[IBIS Ver]   2.1
[File Name]   sprm124.ibs
[File Rev]   0.1
[Date]   Sept. 29, 2003
[Source]   IBIS Model Generated from PACED
[Disclaimer]   Please be aware that in the absence of a written agreement
|   Texas Instruments(TI) assumes no liability for:
|   (1) The accuracy of the IBIS models provided to your company
|   (2) The proper functioning of these Models in your design
|   or for any resulting applications; or
|   (3)Infringement of patents, copyrights or intellectual
|   property rights resulting from your use of these models.
|   TI provides IBIS Models as a service to our customers and
|   therefore reserves the right to limit distribution of the
|   Models.
[Copyright]   Property of Texas Instruments Incorporated.
|   Unauthorized reproduction and/or distribution is strictly.
|   prohibited.
|   This product is protected under copyright law and trade
|   secret law as an unpublished work.
|   Created 1999,(C) Copyright 1999-2000,
|   Texas Instruments Incorporated., All Rights Reserved.
|   These commodities are under the U.S.
|   Government distribution license control. As such,they are
|   not to be re-exported without the prior approval of the U.S.
|   Department of Commerce.
|****** ****   ***** *****   ******  Package Models  **************************
[Component]   6202B_GNY
[Manufacturer]   Texas Instruments
[Package]
|Var   Typ   Min   Max
R_pkg   0.07725   0.03872   0.1717
L_pkg   1.18E-09   5.92E-10   2.62E-09
C_pkg   2.60E-13   1.28E-13   5.40E-13
[Pin]   signal_name   model_name   R_pin   L_pin   C_pin
B10   CLKIN   IDH041   0.0882   2.190E-09   3.140E-13
Y18   CLKOUT1   OUH831   0.0958   2.410E-09   3.560E-13
AB19   CLKOUT2   OUH831   0.1446   3.640E-09   4.900E-13
B12   CLKMODE0   IDH041   0.0766   1.900E-09   2.870E-13
A9   CLKMODE1   IDH041   0.0912   2.250E-09   2.570E-13
A14   CLKMODE2   IDH041   0.0947   2.350E-09   3.390E-13
Y5   TMS   IDH041_PE1001   0.0797   2.000E-09   2.810E-13
AA4   TDO   OUH831   0.1265   3.080E-09   4.160E-13
Y4   TDI   IDH041_PE1001   0.0947   2.270E-09   3.400E-13
AB2   TCK   IDH041_PE1001   0.1540   3.850E-09   4.910E-13
AA3   TRST   IDH041_PE1001   0.1188   2.940E-09   4.230E-13
AA5   EMU1   IDH041_OUH831   0.0985   2.480E-09   3.360E-13
AB4   EMU0   IDH041_OUH831   0.1393   3.510E-09   4.440E-13
J3   RESET   IDH041   0.0624   1.650E-09   2.270E-13
K2   NMI   IDH041   0.0823   2.060E-09   2.810E-13
U2   EXT_INT7   IDH041   0.1088   2.730E-09   3.930E-13
U3   EXT_INT6   IDH041   0.0822   2.080E-09   2.970E-13
W1   EXT_INT5   IDH041   0.1740   4.370E-09   5.930E-13
V2   EXT_INT4   IDH041   0.1390   3.490E-09   5.030E-13
V1   IACK   OUH831   0.1317   3.310E-09   4.520E-13
R3   INUM3   OUH831   0.0685   1.710E-09   2.520E-13
T1   INUM2   OUH831   0.1278   3.220E-09   4.290E-13
T2   INUM1   OUH831   0.0998   2.520E-09   3.310E-13
T3   INUM0   OUH831   0.0772   1.950E-09   2.680E-13
Y2   PD   OUH831   0.1405   3.390E-09   4.000E-13
C8   XCLKIN   IDH041   0.0647   1.620E-09   2.390E-13
A8   XFCLK   OUH831   0.1215   3.050E-09   4.490E-13
C13   XD31   IDH041_OUH831   0.0457   1.130E-09   1.590E-13
A13   XD30   IDH041_OUH831   0.1009   2.520E-09   3.310E-13
C14   XD29   IDH041_OUH831   0.0505   1.260E-09   1.770E-13
B14   XD28   IDH041_OUH831   0.0817   2.010E-09   3.250E-13
B15   XD27   IDH041_OUH831   0.0772   1.920E-09   2.720E-13
C15   XD26   IDH041_OUH831   0.0550   1.370E-09   1.840E-13
A15   XD25   IDH041_OUH831   0.1119   2.830E-09   3.960E-13
B16   XD24   IDH041_OUH831   0.0838   2.080E-09   2.940E-13
C16   XD23   IDH041_OUH831   0.0846   2.110E-09   2.930E-13
A17   XD22   IDH041_OUH831   0.1207   3.000E-09   4.400E-13
B17   XD21   IDH041_OUH831   0.1150   2.960E-09   4.180E-13
C17   XD20   IDH041_OUH831   0.0690   1.710E-09   2.480E-13
B18   XD19   IDH041_OUH831   0.1063   2.640E-09   3.790E-13
A19   XD18   IDH041_OUH831   0.1241   3.170E-09   4.410E-13
C18   XD17   IDH041_OUH831   0.0722   1.790E-09   2.550E-13
B19   XD16   IDH041_OUH831   0.1098   2.740E-09   3.690E-13
C19   XD15   IDH041_OUH831   0.0829   2.060E-09   2.900E-13
B20   XD14   IDH041_OUH831   0.1247   3.120E-09   4.130E-13
A21   XD13   IDH041_OUH831   0.1580   3.980E-09   4.450E-13
C21   XD12   IDH041_OUH831   0.1285   3.260E-09   3.820E-13
D20   XD11   IDH041_OUH831   0.1014   2.550E-09   3.680E-13
B22   XD10   IDH041_OUH831   0.1628   4.130E-09   5.830E-13
D21   XD9   IDH041_OUH831   0.1457   3.650E-09   5.190E-13
E20   XD8   IDH041_OUH831   0.0851   2.140E-09   2.890E-13
E21   XD7   IDH041_OUH831   0.1174   2.940E-09   4.210E-13
D22   XD6   IDH041_OUH831   0.1277   3.240E-09   4.390E-13
F20   XD5   IDH041_OUH831   0.0829   2.070E-09   2.980E-13
F21   XD4   IDH041_OUH831   0.1083   2.700E-09   3.890E-13
E22   XD3   IDH041_OUH831   0.1187   3.000E-09   4.150E-13
G20   XD2   IDH041_OUH831   0.0683   1.710E-09   2.360E-13
G21   XD1   IDH041_OUH831   0.1036   2.600E-09   3.380E-13
G22   XD0   IDH041_OUH831   0.1093   2.830E-09   3.920E-13
D2   XCE3   OUH831   0.1091   2.760E-09   3.830E-13
B1   XCE2   OUH831   0.1584   4.000E-09   5.200E-13
D3   XCE1   OUH831   0.0804   2.040E-09   2.870E-13
C2   XCE0   OUH831   0.0858   2.200E-09   2.520E-13
C5   XBE3/XA5   IDH041_OUH831   0.0844   2.040E-09   3.080E-13
A4   XBE2/XA4   IDH041_OUH831   0.1469   3.700E-09   5.000E-13
B5   XBE1/XA3   IDH041_OUH831   0.1159   2.890E-09   4.470E-13
C6   XBE0/XA2   IDH041_OUH831   0.0820   2.050E-09   3.260E-13
A6   XOE   OUH831   0.1221   3.050E-09   4.570E-13
C7   XRE   OUH831   0.0719   1.810E-09   2.560E-13
B7   XWE/XWAIT   OUH831   0.1011   2.470E-09   3.450E-13
C9   XCS   IDH041   0.0844   2.150E-09   2.860E-13
B6   XAS   IDH041_OUH831   0.1040   2.520E-09   3.750E-13
B9   XCNTL   IDH041   0.0922   2.320E-09   3.310E-13
B8   XW/R   IDH041_OUH831   0.0836   2.030E-09   2.830E-13
C4   XRDY   IDH041_OUH831   0.1205   2.950E-09   4.410E-13
B4   XBLAST   IDH041_OUH831   0.1743   4.390E-09   5.640E-13
A10   XBOFF   IDH041   0.1288   3.220E-09   4.210E-13
A2   XHOLD   IDH041_OUH831   0.1574   3.960E-09   5.380E-13
B3   XHOLDA   IDH041_OUH831   0.1299   3.260E-09   4.720E-13
Y21   CE3   OUH831   0.1187   3.000E-09   3.420E-13
W20   CE2   OUH831   0.0797   2.000E-09   2.830E-13
AA22   CE1   OUH831   0.1873   4.710E-09   5.940E-13
W21   CE0   OUH831   0.1105   2.770E-09   3.800E-13
V20   BE3   OUH831   0.0712   1.790E-09   2.320E-13
V21   BE2   OUH831   0.1055   2.660E-09   3.290E-13
W22   BE1   OUH831   0.1454   3.660E-09   4.520E-13
U20   BE0   OUH831   0.0667   1.660E-09   2.390E-13
H20   EA21   IDH041_OUH831   0.0656   1.620E-09   2.430E-13
H21   EA20   IDH041_OUH831   0.0932   2.310E-09   3.410E-13
H22   EA19   IDH041_OUH831   0.1089   2.800E-09   3.690E-13
J20   EA18   IDH041_OUH831   0.0581   1.460E-09   1.770E-13
J21   EA17   IDH041_OUH831   0.0890   2.250E-09   2.960E-13
K21   EA16   IDH041_OUH831   0.0855   2.120E-09   3.080E-13
K20   EA15   IDH041_OUH831   0.0595   1.470E-09   2.250E-13
K22   EA14   IDH041_OUH831   0.1063   2.630E-09   3.890E-13
L21   EA13   IDH041_OUH831   0.0848   2.100E-09   3.050E-13
L20   EA12   IDH041_OUH831   0.0548   1.350E-09   2.030E-13
L22   EA11   IDH041_OUH831   0.1045   2.600E-09   3.550E-13
M20   EA10   IDH041_OUH831   0.0456   1.130E-09   1.690E-13
M21   EA9   IDH041_OUH831   0.0771   1.910E-09   2.730E-13
N22   EA8   IDH041_OUH831   0.1183   2.940E-09   4.120E-13
N20   EA7   IDH041_OUH831   0.0526   1.310E-09   1.850E-13
N21   EA6   IDH041_OUH831   0.0823   2.060E-09   2.890E-13
P21   EA5   IDH041_OUH831   0.0826   2.070E-09   2.690E-13
P20   EA4   IDH041_OUH831   0.0605   1.540E-09   2.090E-13
R22   EA3   IDH041_OUH831   0.1122   2.800E-09   3.820E-13
R21   EA2   IDH041_OUH831   0.0848   2.100E-09   3.100E-13
Y6   ED31   IDH041_OUH831   0.0620   1.550E-09   2.240E-13
AA6   ED30   IDH041_OUH831   0.0897   2.250E-09   3.310E-13
AB6   ED29   IDH041_OUH831   0.1111   2.790E-09   4.030E-13
Y7   ED28   IDH041_OUH831   0.0620   1.560E-09   2.030E-13
AA7   ED27   IDH041_OUH831   0.0854   2.130E-09   3.040E-13
AB8   ED26   IDH041_OUH831   0.1022   2.540E-09   3.750E-13
Y8   ED25   IDH041_OUH831   0.0503   1.240E-09   1.890E-13
AA8   ED24   IDH041_OUH831   0.0782   1.940E-09   2.760E-13
AA9   ED23   IDH041_OUH831   0.0780   1.940E-09   2.590E-13
Y9   ED22   IDH041_OUH831   0.0504   1.270E-09   1.540E-13
AB10   ED21   IDH041_OUH831   0.1409   3.530E-09   4.740E-13
Y10   ED20   IDH041_OUH831   0.0438   1.080E-09   1.570E-13
AA10   ED19   IDH041_OUH831   0.0683   1.690E-09   2.500E-13
AA11   ED18   IDH041_OUH831   0.0681   1.690E-09   2.380E-13
Y11   ED17   IDH041_OUH831   0.0396   9.690E-10   1.520E-13
AB12   ED16   IDH041_OUH831   0.0934   2.310E-09   3.510E-13
Y12   ED15   IDH041_OUH831   0.0478   1.180E-09   1.770E-13
AA12   ED14   IDH041_OUH831   0.0790   1.960E-09   2.710E-13
AA13   ED13   IDH041_OUH831   0.0999   2.490E-09   3.400E-13
Y13   ED12   IDH041_OUH831   0.0511   1.260E-09   1.860E-13
AB13   ED11   IDH041_OUH831   0.1244   3.130E-09   3.840E-13
Y14   ED10   IDH041_OUH831   0.0862   2.170E-09   2.610E-13
AA14   ED9   IDH041_OUH831   0.0870   2.220E-09   2.930E-13
AA15   ED8   IDH041_OUH831   0.0902   2.280E-09   3.300E-13
Y15   ED7   IDH041_OUH831   0.0662   1.680E-09   2.570E-13
AB15   ED6   IDH041_OUH831   0.1269   3.190E-09   4.740E-13
AA16   ED5   IDH041_OUH831   0.1070   2.700E-09   3.860E-13
Y16   ED4   IDH041_OUH831   0.0852   2.150E-09   3.150E-13
AB17   ED3   IDH041_OUH831   0.1293   3.240E-09   4.800E-13
AA17   ED2   IDH041_OUH831   0.1096   2.750E-09   4.050E-13
Y17   ED1   IDH041_OUH831   0.0864   2.160E-09   3.310E-13
AA18   ED0   IDH041_OUH831   0.1189   2.990E-09   4.180E-13
T21   ARE   OUH831   0.0905   2.270E-09   2.820E-13
R20   AOE   OUH831   0.0603   1.490E-09   2.180E-13
T22   AWE   OUH831   0.1179   2.950E-09   3.920E-13
T20   ARDY   IDH041   0.0645   1.610E-09   2.110E-13
AA19   SDA10   OUH831   0.1546   3.810E-09   5.210E-13
AB21   SDCAS/SSDS   OUH831   0.1670   4.170E-09   4.960E-13
Y19   SDRAS/SSOE   OUH831   0.1075   2.690E-09   3.950E-13
AA20   SDWE/SSWE   OUH831   0.1469   3.620E-09   4.960E-13
V22   HOLD   IDH041   0.1357   3.400E-09   4.260E-13
U21   HOLDA   OUH831   0.0934   2.320E-09   3.330E-13
F2   TOUT1   OUH831   0.0905   2.290E-09   3.290E-13
F3   TINP1   IDH041_PE1001   0.0657   1.670E-09   2.420E-13
D1   TOUT0   OUH831   0.1433   3.650E-09   4.410E-13
E2   TINP0   IDH041   0.1005   2.560E-09   3.520E-13
V3   DMAC3   OUH831   0.1101   2.780E-09   3.860E-13
W2   DMAC2   OUH831   0.1235   3.100E-09   4.600E-13
AA1   DMAC1   OUH831   0.1615   4.060E-09   5.620E-13
W3   DMAC0   OUH831   0.1022   2.590E-09   3.680E-13
K3   CLKS0   IDH041_PE1001   0.0393   9.710E-10   1.430E-13
L2   CLKR0   IDH041_OUH831   0.0771   1.910E-09   2.690E-13
K1   CLKX0   IDH041_OUH831   0.1188   2.960E-09   4.110E-13
M2   DR0   IDH041_PE1001   0.0845   2.100E-09   2.980E-13
M3   DX0   OUH831   0.0429   1.060E-09   1.680E-13
M1   FSR0   IDH041_OUH831   0.1041   2.600E-09   3.540E-13
L3   FSX0   IDH041_OUH831   0.0418   1.030E-09   1.610E-13
E1   CLKS1   IDH041_PE1001   0.1288   3.260E-09   4.190E-13
G2   CLKR1   IDH041_OUH831   0.0887   2.250E-09   3.090E-13
G3   CLKX1   IDH041_OUH831   0.0629   1.590E-09   2.360E-13
H1   DR1   IDH041_PE1001   0.0886   2.220E-09   3.130E-13
H2   DX1   OUH831   0.0838   2.100E-09   3.090E-13
H3   FSR1   IDH041_OUH831   0.0762   2.030E-09   2.830E-13
G1   FSX1   IDH041_OUH831   0.1162   2.940E-09   3.880E-13
N1   CLKS2   IDH041_PE1001   0.1059   2.630E-09   3.900E-13
N2   CLKR2   IDH041_OUH831   0.0899   2.240E-09   3.180E-13
N3   CLKX2   IDH041_OUH831   0.0553   1.370E-09   2.090E-13
R2   DR2   IDH041_PE1001   0.0924   2.290E-09   3.370E-13
R1   DX2   IDH041_OUH831   0.1162   2.900E-09   3.970E-13
P3   FSR2   IDH041_OUH831   0.0642   1.610E-09   1.960E-13
P2   FSX2   IDH041_OUH831   0.0902   2.260E-09   2.940E-13
[Component]   6202B_GNZ
[Manufacturer]   Texas Instruments
[Package]
|Var   Typ   Min   Max
R_pkg   0.3219   0.02687   0.5697
L_pkg   6.28E-09   4.21E-10   1.09E-08
C_pkg   6.05E-13   3.91E-14   1.19E-12
[Pin]   signal_name model_name   R_pin   L_pin   C_pin
C12   CLKIN   IDH041   0.2638   4.990E-09   4.910E-13
AD20   CLKOUT1   OUH831   0.2991   5.950E-09   5.810E-13
AC19   CLKOUT2   OUH831   0.2057   4.080E-09   3.900E-13
B15   CLKMODE0   IDH041   0.3116   5.970E-09   6.150E-13
C11   CLKMODE1   IDH041   0.2621   5.060E-09   4.900E-13
AD7   TMS   IDH041_PE1001   0.3561   7.170E-09   7.110E-13
AE6   TDO   OUH831   0.4907   9.610E-09   9.780E-13
AF5   TDI   IDH041_PE1001   0.5372   1.060E-08   1.010E-12
AE5   TCK   IDH041_PE1001   0.4052   8.240E-09   7.460E-13
AC7   TRST   IDH041_PE1001   0.3029   6.050E-09   6.360E-13
AF6   EMU1   IDH041_OUH831   0.5054   1.000E-08   9.090E-13
AC8   EMU0   IDH041_OUH831   0.3024   6.120E-09   6.080E-13
K2   RESET   IDH041   0.3503   6.760E-09   6.610E-13
L2   NMI   IDH041   0.3382   6.510E-09   6.060E-13
V4   EXT_INT7   IDH041   0.1645   3.180E-09   3.280E-13
Y2   EXT_INT6   IDH041   0.2400   4.890E-09   4.610E-13
AA1   EXT_INT5   IDH041   0.4222   8.210E-09   7.890E-13
W4   EXT_INT4   IDH041   0.2400   4.890E-09   4.610E-13
Y1   IACK   OUH831   0.2400   4.890E-09   4.610E-13
V2   INUM3   OUH831   0.3081   5.920E-09   5.130E-13
U4   INUM2   OUH831   0.1917   3.670E-09   3.750E-13
V3   INUM1   OUH831   0.2469   4.770E-09   4.480E-13
W2   INUM0   OUH831   0.3115   6.010E-09   5.600E-13
AB2   PD   OUH831   0.3340   6.580E-09   5.950E-13
A9   XCLKIN   IDH041   0.3536   6.900E-09   5.980E-13
B9   XFCLK   OUH831   0.2805   5.470E-09   5.180E-13
D15   XD31   IDH041_OUH831   0.1719   3.250E-09   3.080E-13
B16   XD30   IDH041_OUH831   0.2810   5.500E-09   4.950E-13
A17   XD29   IDH041_OUH831   0.3570   6.870E-09   6.200E-13
B17   XD28   IDH041_OUH831   0.3263   6.320E-09   5.960E-13
D16   XD27   IDH041_OUH831   0.2076   4.030E-09   4.140E-13
A18   XD26   IDH041_OUH831   0.3553   6.920E-09   6.280E-13
B18   XD25   IDH041_OUH831   0.3073   6.010E-09   5.500E-13
D17   XD24   IDH041_OUH831   0.1879   3.720E-09   3.630E-13
C18   XD23   IDH041_OUH831   0.2796   5.480E-09   5.520E-13
A20   XD22   IDH041_OUH831   0.4213   8.230E-09   7.210E-13
D18   XD21   IDH041_OUH831   0.2194   4.360E-09   4.440E-13
C19   XD20   IDH041_OUH831   0.2924   5.780E-09   5.640E-13
A21   XD19   IDH041_OUH831   0.4309   8.490E-09   7.490E-13
D19   XD18   IDH041_OUH831   0.2326   4.670E-09   4.520E-13
C20   XD17   IDH041_OUH831   0.2855   5.590E-09   5.870E-13
B21   XD16   IDH041_OUH831   0.4291   8.460E-09   8.410E-13
A22   XD15   IDH041_OUH831   0.4723   9.200E-09   9.000E-13
D20   XD14   IDH041_OUH831   0.2354   4.750E-09   5.000E-13
B22   XD13   IDH041_OUH831   0.3685   7.380E-09   6.440E-13
E25   XD12   IDH041_OUH831   0.3874   7.630E-09   6.650E-13
F24   XD11   IDH041_OUH831   0.3659   7.170E-09   7.210E-13
E26   XD10   IDH041_OUH831   0.5044   9.790E-09   1.010E-12
F25   XD9   IDH041_OUH831   0.4704   9.110E-09   9.340E-13
G24   XD8   IDH041_OUH831   0.3067   5.990E-09   6.270E-13
H23   XD7   IDH041_OUH831   0.2528   4.930E-09   4.760E-13
F26   XD6   IDH041_OUH831   0.4563   8.810E-09   8.540E-13
G25   XD5   IDH041_OUH831   0.3770   7.300E-09   6.950E-13
J23   XD4   IDH041_OUH831   0.2358   4.580E-09   4.770E-13
G26   XD3   IDH041_OUH831   0.4407   8.520E-09   8.090E-13
H25   XD2   IDH041_OUH831   0.3722   7.200E-09   6.880E-13
J24   XD1   IDH041_OUH831   0.3026   5.860E-09   5.680E-13
K23   XD0   IDH041_OUH831   0.2403   4.650E-09   4.790E-13
F2   XCE3   OUH831   0.4601   9.080E-09   9.240E-13
E1   XCE2   OUH831   0.4955   9.760E-09   1.010E-12
F3   XCE1   OUH831   0.3550   7.130E-09   7.310E-13
E2   XCE0   OUH831   0.3747   7.520E-09   6.670E-13
C7   XBE3/XA5   IDH041_OUH831   0.2845   5.590E-09   5.770E-13
D8   XBE2/XA4   IDH041_OUH831   0.2296   4.610E-09   4.450E-13
A6   XBE1/XA3   IDH041_OUH831   0.4322   8.490E-09   7.670E-13
C8   XBE0/XA2   IDH041_OUH831   0.2893   5.720E-09   5.510E-13
A7   XOE   OUH831   0.4201   8.180E-09   7.130E-13
C9   XRE   OUH831   0.2770   5.420E-09   5.390E-13
D10   XWE/XWAIT   OUH831   0.1839   3.620E-09   3.570E-13
A10   XCS   IDH041   0.3575   6.830E-09   6.400E-13
D9   XAS   IDH041_OUH831   0.2189   4.310E-09   4.370E-13
B10   XCNTL   IDH041   0.3317   6.410E-09   5.970E-13
D11   XW/R   IDH041_OUH831   0.2027   3.920E-09   4.050E-13
A5   XRDY   IDH041_OUH831   0.4729   9.180E-09   8.950E-13
B6   XBLAST   IDH041_OUH831   0.4320   8.500E-09   8.260E-13
B11   XBOFF   IDH041   0.2772   5.340E-09   5.080E-13
B5   XHOLD   IDH041_OUH831   0.3669   7.320E-09   6.340E-13
D7   XHOLDA   IDH041_OUH831   0.2321   4.690E-09   4.990E-13
AB25   CE3   OUH831   0.3742   7.580E-09   6.740E-13
AA24   CE2   OUH831   0.3517   7.120E-09   7.300E-13
AB26   CE1   OUH831   0.4918   9.750E-09   1.010E-12
AA25   CE0   OUH831   0.4564   9.080E-09   9.020E-13
Y24   BE3   OUH831   0.2400   4.890E-09   4.610E-13
W23   BE2   OUH831   0.2400   4.890E-09   4.610E-13
AA26   BE1   OUH831   0.4404   8.720E-09   8.160E-13
Y25   BE0   OUH831   0.2400   4.890E-09   4.610E-13
J25   EA21   IDH041_OUH831   0.3504   6.790E-09   6.080E-13
J26   EA20   IDH041_OUH831   0.4034   7.770E-09   7.340E-13
L23   EA19   IDH041_OUH831   0.2252   4.330E-09   4.500E-13
K25   EA18   IDH041_OUH831   0.3499   6.750E-09   6.280E-13
L24   EA17   IDH041_OUH831   0.2829   5.450E-09   5.510E-13
L25   EA16   IDH041_OUH831   0.3382   6.500E-09   6.080E-13
M23   EA15   IDH041_OUH831   0.2183   4.180E-09   3.710E-13
M24   EA14   IDH041_OUH831   0.2689   5.140E-09   5.380E-13
M25   EA13   IDH041_OUH831   0.3728   7.110E-09   7.000E-13
N23   EA12   IDH041_OUH831   0.4099   7.780E-09   8.420E-13
P24   EA11   IDH041_OUH831   0.3313   6.340E-09   6.780E-13
P23   EA10   IDH041_OUH831   0.4650   8.830E-09   1.040E-12
R25   EA9   IDH041_OUH831   0.3734   7.150E-09   7.250E-13
R24   EA8   IDH041_OUH831   0.3206   6.150E-09   6.370E-13
R23   EA7   IDH041_OUH831   0.2651   5.090E-09   4.740E-13
T25   EA6   IDH041_OUH831   0.3378   6.510E-09   5.940E-13
T24   EA5   IDH041_OUH831   0.2870   5.550E-09   5.260E-13
U25   EA4   IDH041_OUH831   0.3343   6.450E-09   6.200E-13
T23   EA3   IDH041_OUH831   0.2251   4.380E-09   4.570E-13
V26   EA2   IDH041_OUH831   0.4146   8.080E-09   7.390E-13
AD8   ED31   IDH041_OUH831   0.3680   7.360E-09   7.280E-13
AC9   ED30   IDH041_OUH831   0.3096   6.220E-09   6.420E-13
AF7   ED29   IDH041_OUH831   0.5081   1.000E-08   8.990E-13
AD9   ED28   IDH041_OUH831   0.3801   7.620E-09   6.780E-13
AC10   ED27   IDH041_OUH831   0.2208   4.350E-09   4.270E-13
AE9   ED26   IDH041_OUH831   0.3326   6.490E-09   5.910E-13
AF9   ED25   IDH041_OUH831   0.3858   7.480E-09   6.920E-13
AC11   ED24   IDH041_OUH831   0.2097   4.080E-09   4.190E-13
AE10   ED23   IDH041_OUH831   0.3226   6.270E-09   5.930E-13
AD11   ED22   IDH041_OUH831   0.2625   5.150E-09   4.870E-13
AE11   ED21   IDH041_OUH831   0.3179   6.200E-09   5.610E-13
AC12   ED20   IDH041_OUH831   0.2012   3.870E-09   3.780E-13
AD12   ED19   IDH041_OUH831   0.2534   4.860E-09   4.780E-13
AE12   ED18   IDH041_OUH831   0.3579   6.820E-09   6.970E-13
AC13   ED17   IDH041_OUH831   0.1961   3.780E-09   3.730E-13
AD14   ED16   IDH041_OUH831   0.3163   6.130E-09   5.910E-13
AC14   ED15   IDH041_OUH831   0.2550   4.920E-09   5.040E-13
AE15   ED14   IDH041_OUH831   0.3636   6.980E-09   6.820E-13
AD15   ED13   IDH041_OUH831   0.3111   5.980E-09   6.110E-13
AC15   ED12   IDH041_OUH831   0.2527   4.870E-09   4.870E-13
AE16   ED11   IDH041_OUH831   0.3246   6.270E-09   5.810E-13
AD16   ED10   IDH041_OUH831   0.2710   5.230E-09   4.800E-13
AE17   ED9   IDH041_OUH831   0.3284   6.340E-09   6.220E-13
AC16   ED8   IDH041_OUH831   0.2116   4.110E-09   4.230E-13
AF18   ED7   IDH041_OUH831   0.3892   7.540E-09   7.000E-13
AE18   ED6   IDH041_OUH831   0.3365   6.550E-09   5.870E-13
AC17   ED5   IDH041_OUH831   0.2262   4.430E-09   4.440E-13
AD18   ED4   IDH041_OUH831   0.2828   5.550E-09   5.270E-13
AF20   ED3   IDH041_OUH831   0.4191   8.190E-09   7.040E-13
AC18   ED2   IDH041_OUH831   0.2280   4.490E-09   4.610E-13
AD19   ED1   IDH041_OUH831   0.2904   5.730E-09   5.470E-13
AF21   ED0   IDH041_OUH831   0.4335   8.500E-09   7.440E-13
V24   ARE   OUH831   0.2894   5.770E-09   5.390E-13
V25   AOE   OUH831   0.3356   6.550E-09   5.890E-13
U23   AWE   OUH831   0.2349   4.630E-09   4.800E-13
W25   ARDY   IDH041   0.2400   4.890E-09   4.610E-13
AE21   SDA10   OUH831   0.3780   7.320E-09   7.490E-13
AE22   SDCAS/SSDS  OUH831   0.4007   7.940E-09   6.670E-13
AF22   SDRAS/SSOE  OUH831   0.4133   7.980E-09   7.820E-13
AC20   SDWE/SSWE   OUH831   0.2341   4.690E-09   5.010E-13
Y26   HOLD   IDH041   0.2400   4.890E-09   4.610E-13
V23   HOLDA   OUH831   0.2255   4.530E-09   4.730E-13
J4   TOUT1   OUH831   0.2740   5.410E-09   5.710E-13
G2   TINP1   IDH041_PE1001   0.3678   7.280E-09   6.790E-13
F1   TOUT0   OUH831   0.4424   8.720E-09   8.180E-13
H4   TINP0   IDH041   0.2435   4.910E-09   4.620E-13
Y3   DMAC3   OUH831   0.2400   4.890E-09   4.610E-13
AA2   DMAC2   OUH831   0.4274   8.370E-09   8.540E-13
AB1   DMAC1   OUH831   0.4511   8.830E-09   9.040E-13
AA3   DMAC0   OUH831   0.3099   6.120E-09   6.190E-13
M4   CLKS0   IDH041_PE1001   0.2747   5.190E-09   4.900E-13
M2   CLKR0   IDH041_OUH831   0.3215   6.170E-09   5.830E-13
M3   CLKX0   IDH041_OUH831   0.2058   3.890E-09   3.540E-13
R2   DR0   IDH041_PE1001   0.2836   5.420E-09   5.010E-13
P4   DX0   OUH831   0.0269   4.210E-10   3.910E-14
N3   FSR0   IDH041_OUH831   0.3111   6.000E-09   5.040E-13
N4   FSX0   IDH041_OUH831   0.0453   8.050E-10   8.610E-14
G1   CLKS1   IDH041_PE1001   0.4882   9.490E-09   9.240E-13
J3   CLKR1   IDH041_OUH831   0.2935   5.780E-09   5.520E-13
H2   CLKX1   IDH041_OUH831   0.4171   8.120E-09   8.170E-13
L4   DR1   IDH041_PE1001   0.2274   4.390E-09   4.560E-13
J1   DX1   OUH831   0.3961   7.750E-09   7.370E-13
J2   FSR1   IDH041_OUH831   0.3465   6.780E-09   6.100E-13
K4   FSX1   IDH041_OUH831   0.2367   4.640E-09   4.820E-13
R3   CLKS2   IDH041_PE1001   0.2174   4.080E-09   3.890E-13
T2   CLKR2   IDH041_OUH831   0.3068   5.870E-09   5.320E-13
R4   CLKX2   IDH041_OUH831   0.2146   4.010E-09   3.450E-13
V1   DR2   IDH041_PE1001   0.3534   6.790E-09   6.270E-13
T4   DX2   IDH041_OUH831   0.1817   3.450E-09   3.580E-13
U2   FSR2   IDH041_OUH831   0.3139   6.000E-09   5.430E-13
T3   FSX2   IDH041_OUH831   0.2631   4.930E-09   4.960E-13
| End of package information
| Models and submodels in the file (4): IDH041 (Input), IDH041_PE1001 (Input), OUH831 (3-state), IDH041_OUH831 (I/O)
